| IBIS file stm32l4r5_s5_r7_s7_lqfp100.ibs
[IBIS ver]   4.2
[File name]   stm32l4r5_s5_r7_s7_lqfp100.ibs
[File Rev]   1.0
[Date]   01-6-2017
[Source]   Data Created at STMicroelectronics
[Notes]   File originated from ELDO simulations.
[Disclaimer]  This information is for modeling purpose only and is
   not guaranted.
   The information is subject to change without notice.
[Copyright]   Copyright 2017 STMicroelectronics Inc.
|   Component stm32l4r5_s5_r7_s7_lqfp100
[Component] stm32l4r5_s5_r7_s7_lqfp100
[Manufacturer] STMicroelectronics
[Package]
| variable   typ   min   max
R_pkg   0.0   0.0   0.0
L_pkg   0.0H   0.0H   0.0H
C_pkg   0.0F   0.0F   0.0F
[Pin]  signal_name   model_name   R_pin   L_pin   C_pin
1 PE2 io8prog2m25m50m120m_sudq_ft 132.430E-3 7.034E-9 135.000E-15
2 PE3 io8prog2m25m50m120m_sudq_ft 133.348E-3 6.765E-9 19.500E-15
3 PE4 io8prog2m25m50m120m_sudq_ft 128.973E-3 6.495E-9 10.400E-15
4 PE5 io8prog2m25m50m120m_sudq_ft 125.345E-3 6.206E-9 5.240E-15
5 PE6 io8prog2m25m50m120m_sudq_ft 120.515E-3 5.991E-9 7.820E-15
6 VBAT power 120.471E-3 5.950E-9 6.530E-15
7 PC13 io8prog2m25m50m120m_sudq_ft 117.881E-3 5.783E-9 6.230E-15
8 PC14-OSC32_IN io8prog2m25m50m120m_sudq_ft 117.279E-3 5.654E-9 3.110E-15
9 PC15-OSC32_OUT io8prog2m25m50m120m_sudq_ft 115.548E-3 5.548E-9 1.390E-15
10 VSS gnd 114.996E-3 5.434E-9 2.920E-15
11 VDD power 112.976E-3 5.296E-9 3.560E-15
12 PH0-OSC_IN io8prog2m25m50m120m_sudq_ft 111.323E-3 5.231E-9 4.780E-15
13 PH1-OSC_OUT io8prog2m25m50m120m_sudq_ft 109.217E-3 5.142E-9 8.660E-15
14 NRST ioreset_ft_v33 110.664E-3 5.180E-9 9.030E-15
15 PC0 io8prog2m25m50m120m_sudq_i2c_ft 110.608E-3 5.192E-9 7.980E-15
16 PC1 io8prog2m25m50m120m_sudq_i2c_ft 111.326E-3 5.252E-9 10.300E-15
17 PC2 io8prog2m25m50m120m_sudq_ft 114.420E-3 5.345E-9 7.000E-15
18 PC3 io8prog2m25m50m120m_sudq_ft 114.363E-3 5.454E-9 8.650E-15
19 VSSA gnd 117.564E-3 5.621E-9 7.825E-15
20 VREF- gnd 119.905E-3 5.800E-9 229.000E-18
21 VREF+ power 122.312E-3 5.963E-9 1.050E-15
22 VDDA power 125.384E-3 6.187E-9 812.000E-18
23 PA0 io8prog2m25m50m120m_sudq_ft 129.702E-3 6.485E-9 3.820E-15
24 PA1 io8prog2m25m50m120m_sudq_ft 132.290E-3 6.715E-9 6.800E-15
25 PA2 io8prog2m25m50m120m_sudq_ft 132.955E-3 7.014E-9 16.700E-15
26 PA3 io8prog2m25m50m120m_sudq_ft 133.943E-3 7.050E-9 17.500E-15
27 VSS gnd 134.958E-3 6.804E-9 12.700E-15
28 VDD power 130.511E-3 6.528E-9 9.830E-15
29 PA4 io8prog2m25m50m120m_sudq_ft 125.387E-3 6.245E-9 6.070E-15
30 PA5 io8prog2m25m50m120m_sudq_ft 124.989E-3 6.108E-9 577.000E-18
31 PA6 io8prog2m25m50m120m_sudq_ft 121.784E-3 5.890E-9 1.520E-15
32 PA7 io8prog2m25m50m120m_sudq_i2c_ft 119.149E-3 5.716E-9 5.440E-15
33 PC4 io8prog2m25m50m120m_sudq_ft 116.375E-3 5.556E-9 4.100E-15
34 PC5 io8prog2m25m50m120m_sudq_ft 113.279E-3 5.415E-9 3.690E-15
35 PB0 io8prog2m25m50m120m_sudq_ft 112.727E-3 5.358E-9 3.895E-15
36 PB1 io8prog2m25m50m120m_sudq_ft 112.271E-3 5.272E-9 1.660E-15
37 PB2 io8prog2m25m50m120m_sudq_ft 111.816E-3 5.238E-9 7.920E-15
38 PE7 io8prog2m25m50m120m_sudq_ft 110.999E-3 5.184E-9 9.900E-15
39 PE8 io8prog2m25m50m120m_sudq_ft 114.589E-3 5.299E-9 7.910E-15
40 PE9 io8prog2m25m50m120m_sudq_ft 114.461E-3 5.333E-9 7.940E-15
41 PE10 io8prog2m25m50m120m_sudq_ft 115.350E-3 5.424E-9 4.180E-15
42 PE11 io8prog2m25m50m120m_sudq_ft 116.979E-3 5.533E-9 6.060E-15
43 PE12 io8prog2m25m50m120m_sudq_ft 120.185E-3 5.698E-9 5.120E-15
44 PE13 io8prog2m25m50m120m_sudq_ft 122.587E-3 5.871E-9 4.740E-15
45 PE14 io8prog2m25m50m120m_sudq_ft 126.303E-3 6.069E-9 11.600E-15
46 PE15 io8prog2m25m50m120m_sudq_ft 129.715E-3 6.277E-9 9.910E-15
47 PB10 io8prog2m25m50m120m_sudq_i2c_ft 133.373E-3 6.508E-9 5.080E-15
48 PB11 io8prog2m25m50m120m_sudq_i2c_ft 137.888E-3 6.857E-9 5.470E-15
49 VSS gnd 131.554E-3 6.802E-9 4.180E-15
50 VDD power 132.348E-3 7.042E-9 11.900E-15
51 PB12 io8prog2m25m50m120m_sudq_ft 131.768E-3 7.008E-9 16.200E-15
52 PB13 io8prog2m25m50m120m_sudq_i2c_ft 131.784E-3 6.751E-9 2.150E-15
53 PB14 io8prog2m25m50m120m_sudq_i2c_ft 129.151E-3 6.483E-9 9.175E-15
54 PB15 io8prog2m25m50m120m_sudq_ft 125.191E-3 6.202E-9 5.663E-15
55 PD8 io8prog2m25m50m120m_sudq_ft 121.530E-3 5.986E-9 3.690E-15
56 PD9 io8prog2m25m50m120m_sudq_ft 118.874E-3 5.807E-9 7.430E-15
57 PD10 io8prog2m25m50m120m_sudq_ft 115.870E-3 5.635E-9 10.600E-15
58 PD11 io8prog2m25m50m120m_sudq_ft 113.226E-3 5.471E-9 5.760E-15
59 PD12 io8prog2m25m50m120m_sudq_ft 111.782E-3 5.354E-9 6.530E-15
60 PD13 io8prog2m25m50m120m_sudq_ft 110.713E-3 5.276E-9 11.400E-15
61 PD14 io8prog2m25m50m120m_sudq_ft 110.052E-3 5.204E-9 13.200E-15
62 PD15 io8prog2m25m50m120m_sudq_ft 109.954E-3 5.180E-9 14.600E-15
63 PC6 io8prog2m25m50m120m_sudq_ft 109.780E-3 5.154E-9 7.250E-15
64 PC7 io8prog2m25m50m120m_sudq_ft 112.446E-3 5.258E-9 359.000E-18
65 PC8 io8prog2m25m50m120m_sudq_ft 113.596E-3 5.332E-9 658.000E-18
66 PC9 io8prog2m25m50m120m_sudq_ft 115.707E-3 5.466E-9 508.500E-18
67 PA8 io8prog2m25m50m120m_sudq_ft 116.952E-3 5.598E-9 583.250E-18
68 PA9 power 119.043E-3 5.762E-9 545.875E-18
69 PA10 io8usb_id_otg20_lcd4_ft_ms 120.674E-3 5.880E-9 13.900E-15
70 PA11 io8usblsfs_otg2 124.659E-3 6.108E-9 25.000E-15
71 PA12 io8usblsfs_otg2 124.407E-3 6.161E-9 39.900E-15
72 PA13 io8prog2m25m50m120m_sudq_ft 130.156E-3 6.404E-9 302.000E-15
73 VDDUSB power 135.110E-3 6.824E-9 155.000E-15
74 VSS gnd 139.402E-3 7.077E-9 155.000E-15
75 VDD gnd 133.554E-3 7.056E-9 39.000E-15
76 PA14 io8prog2m25m50m120m_sudq_ft 135.295E-3 7.104E-9 16.300E-15
77 PA15 io8prog2m25m50m120m_sudq_ft 132.514E-3 6.836E-9 9.760E-15
78 PC10 io8prog2m25m50m120m_sudq_ft 133.482E-3 6.641E-9 9.300E-15
79 PC11 io8prog2m25m50m120m_sudq_ft 128.366E-3 6.341E-9 5.420E-15
80 PC12 io8prog2m25m50m120m_sudq_ft 124.282E-3 6.092E-9 1.180E-15
81 PD0 io8prog2m25m50m120m_sudq_ft 121.841E-3 5.917E-9 5.460E-15
82 PD1 io8prog2m25m50m120m_sudq_ft 118.487E-3 5.728E-9 7.000E-15
83 PD2 io8prog2m25m50m120m_sudq_ft 117.180E-3 5.573E-9 6.060E-15
84 PD3 io8prog2m25m50m120m_sudq_ft 113.501E-3 5.422E-9 5.450E-15
85 PD4 io8prog2m25m50m120m_sudq_ft 113.789E-3 5.344E-9 529.000E-18
86 PD5 io8prog2m25m50m120m_sudq_ft 110.806E-3 5.256E-9 2.990E-15
87 PD6 io8prog2m25m50m120m_sudq_ft 110.442E-3 5.246E-9 2.060E-15
88 PD7 io8prog2m25m50m120m_sudq_ft 111.525E-3 5.178E-9 5.680E-15
89 PB3 io8prog2m25m50m120m_sudq_ft 111.144E-3 5.223E-9 9.910E-15
90 PB4 io8prog2m25m50m120m_sudq_i2c_ft 113.222E-3 5.310E-9 9.050E-15
91 PB5 io8prog2m25m50m120m_sudq_ft 113.323E-3 5.401E-9 12.900E-15
92 PB6 io8prog2m25m50m120m_sudq_i2c_ft 115.849E-3 5.519E-9 12.600E-15
93 PB7 io8prog2m25m50m120m_sudq_i2c_ft 117.578E-3 5.673E-9 6.140E-15
94 PH3-BOOT0 io8prog2m25m50m120m_sudq_ft 118.982E-3 5.802E-9 9.370E-15
95 PB8 io8prog2m25m50m120m_sudq_i2c_ft 121.886E-3 5.962E-9 7.755E-15
96 PB9 io8prog2m25m50m120m_sudq_i2c_ft 126.276E-3 6.158E-9 8.563E-15
97 PE0 io8prog2m25m50m120m_sudq_ft 128.749E-3 6.367E-9 8.159E-15
98 PE1 io8prog2m25m50m120m_sudq_ft 133.288E-3 6.700E-9 1.030E-15
99 VSS gnd 132.230E-3 6.844E-9 4.410E-15
100 VDD power 132.277E-3 7.052E-9 17.100E-15
[Diff Pin]   inv_pin   vdiff   tdelay_typ  tdelay_min  tdelay_max
70 71 200mV   NA   NA   NA
[Model Selector] io8prog2m25m50m120m_sudq_ft
io8p00_sudq_ft_pd_lv  "SPEED00, PD=40kOhm - 1P8V"
io8p00_sudq_ft_pu_lv  "SPEED00, PU=40kOhm - 1P8V"
io8p00_sudq_ft_lv  "SPEED00 - 1P8V"
io8p00_sudq_ft_pd  "SPEED00, PD=40kOhm - 3P3V"
io8p00_sudq_ft_pu  "SPEED00, PU=40kOhm - 3P3V"
io8p00_sudq_ft  "SPEED00 - 3P3V"
io8p01_sudq_ft_pd_lv  "SPEED01, PD=40kOhm - 1P8V"
io8p01_sudq_ft_pu_lv  "SPEED01, PU=40kOhm - 1P8V"
io8p01_sudq_ft_lv  "SPEED01 - 1P8V"
io8p01_sudq_ft_pd  "SPEED01, PD=40kOhm - 3P3V"
io8p01_sudq_ft_pu  "SPEED01, PU=40kOhm - 3P3V"
io8p01_sudq_ft  "SPEED01 - 3P3V"
io8p10_sudq_ft_pd_lv  "SPEED10, PD=40kOhm - 1P8V"
io8p10_sudq_ft_pu_lv  "SPEED10, PU=40kOhm - 1P8V"
io8p10_sudq_ft_lv  "SPEED10 - 1P8V"
io8p10_sudq_ft_pd  "SPEED10, PD=40kOhm - 3P3V"
io8p10_sudq_ft_pu  "SPEED10, PU=40kOhm - 3P3V"
io8p10_sudq_ft  "SPEED10 - 3P3V"
io8p11_sudq_ft_pd_lv  "SPEED11, PD=40kOhm - 1P8V"
io8p11_sudq_ft_pu_lv  "SPEED11, PU=40kOhm - 1P8V"
io8p11_sudq_ft_lv  "SPEED11 - 1P8V"
io8p11_sudq_ft_pd  "SPEED11, PD=40kOhm - 3P3V"
io8p11_sudq_ft_pu  "SPEED11, PU=40kOhm - 3P3V"
io8p11_sudq_ft  "SPEED11 - 3P3V"
[Model Selector] io8prog2m25m50m120m_sudq_i2c_ft
io8prog_1v8_i2c_pd  "5V Tol GPIO 1.8V range i2c functionality with pull down"
io8prog_1v8_i2c_pu  "5V Tol GPIO 1.8V range i2c functionality with pull up"
io8prog_1v8_i2c  "5V Tol GPIO 1.8V range i2c functionality"
io8prog_3v3_i2c_pd  "5V Tol GPIO 3.3V range i2c functionality with pull down"
io8prog_3v3_i2c_pu  "5V Tol GPIO 3.3V range i2c functionality with pull up"
io8prog_3v3_i2c  "5V Tol GPIO 3.3V range i2c functionality"
io8prog_1v8_pd_00  "5V Tol GPIO 1.8V range with pd speed 00"
io8prog_1v8_pu_00  "5V Tol GPIO 1.8V range with pu speed 00"
io8prog_1v8_00  "5V Tol GPIO 1.8V range speed 00"
io8prog_3v3_pd_00  "5V Tol GPIO 3.3V range with pd speed 00"
io8prog_3v3_pu_00  "5V Tol GPIO 3.3V range with pu speed 00"
io8prog_3v3_00  "5V Tol GPIO 3.3V range speed 00"
io8prog_1v8_pd_01  "5V Tol GPIO 1.8V range with pd speed 01"
io8prog_1v8_pu_01  "5V Tol GPIO 1.8V range with pu speed 01"
io8prog_1v8_01  "5V Tol GPIO 1.8V range speed 01"
io8prog_3v3_pd_01  "5V Tol GPIO 3.3V range with pd speed 01"
io8prog_3v3_pu_01  "5V Tol GPIO 3.3V range with pu speed 01"
io8prog_3v3_01  "5V Tol GPIO 3.3V range speed 01"
io8prog_1v8_pd_10  "5V Tol GPIO 1.8V range with pd speed 10"
io8prog_1v8_pu_10  "5V Tol GPIO 1.8V range with pu speed 10"
io8prog_1v8_10  "5V Tol GPIO 1.8V range speed 10"
io8prog_3v3_pd_10  "5V Tol GPIO 3.3V range with pd speed 10"
io8prog_3v3_pu_10  "5V Tol GPIO 3.3V range with pu speed 10"
io8prog_3v3_10  "5V Tol GPIO 3.3V range speed 10"
io8prog_1v8_pd_11  "5V Tol GPIO 1.8V range with pd speed 11"
io8prog_1v8_pu_11  "5V Tol GPIO 1.8V range with pu speed 11"
io8prog_1v8_11  "5V Tol GPIO 1.8V range speed 11"
io8prog_3v3_pd_11  "5V Tol GPIO 3.3V range with pd speed 11"
io8prog_3v3_pu_11  "5V Tol GPIO 3.3V range with pu speed 11"
io8prog_3v3_11  "5V Tol GPIO 3.3V range speed 11"
[Model Selector] io8usb_id_otg20_lcd4_ft_ms
io8usbid_1v8_id_pu  "ID 1V8 range with pull up"
io8usbid_3v3_id_pu  "ID 3V3 range with pull up"
io8usbid_1v8_id  "ID 1V8 range"
io8usbid_3v3_id  "ID 3V3 range"
io8usbid_1v8_pd_00  "GPIO 1.8V range with pd speed 00"
io8usbid_1v8_pu_00  "GPIO 1.8V range with pu speed 00"
io8usbid_1v8_00  "GPIO 1.8V range speed 00"
io8usbid_3v3_pd_00  "GPIO 3.3V range with pd speed 00"
io8usbid_3v3_pu_00  "GPIO 3.3V range with pu speed 00"
io8usbid_3v3_00  "GPIO 3.3V range speed 00"
io8usbid_1v8_pd_01  "GPIO 1.8V range with pd speed 01"
io8usbid_1v8_pu_01  "GPIO 1.8V range with pu speed 01"
io8usbid_1v8_01  "GPIO 1.8V range speed 01"
io8usbid_3v3_pd_01  "GPIO 3.3V range with pd speed 01"
io8usbid_3v3_pu_01  "GPIO 3.3V range with pu speed 01"
io8usbid_3v3_01  "GPIO 3.3V range speed 01"
io8usbid_1v8_pd_10  "GPIO 1.8V range with pd speed 10"
io8usbid_1v8_pu_10  "GPIO 1.8V range with pu speed 10"
io8usbid_1v8_10  "GPIO 1.8V range speed 10"
io8usbid_3v3_pd_10  "GPIO 3.3V range with pd speed 10"
io8usbid_3v3_pu_10  "GPIO 3.3V range with pu speed 10"
io8usbid_3v3_10  "GPIO 3.3V range speed 10"
io8usbid_1v8_pd_11  "GPIO 1.8V range with pd speed 11"
io8usbid_1v8_pu_11  "GPIO 1.8V range with pu speed 11"
io8usbid_1v8_11  "GPIO 1.8V range speed 11"
io8usbid_3v3_pd_11  "GPIO 3.3V range with pd speed 11"
io8usbid_3v3_pu_11  "GPIO 3.3V range with pu speed 11"
io8usbid_3v3_11  "GPIO 3.3V range speed 11"
[Model Selector] io8usblsfs_otg2
usb_ls_pd  "USB Low Speed mode - Pull Down"
usb_ls_pu2  "USB Low Speed mode - Pull up 2"
usb_ls_pu  "USB Low Speed mode - Pull up"
usb_fs  "USB Low Speed mode"
usb_fs_pd  "USB Full Speed mode - Pull Down"
usb_fs_pu2  "USB Full Speed mode - Pull up 2"
usb_fs_pu  "USB Full Speed mode - Pull up"
[Model Selector] ioreset_ft_v33
ioreset_1v2_pu  "RESET 1.2V range with PU"
ioreset_1v2  "RESET 1.2V range"
ioreset_1v8_pu  "RESET 1.8V range with PU"
ioreset_1v8  "RESET 1.8V range"
ioreset_3v3_pu  "RESET 3.3V range with PU"
ioreset_3v3  "RESET 3.3V range"
| Models and submodels in the file (95): io8p00_sudq_ft_pd_lv (I/O), io8p00_sudq_ft_pu_lv (I/O), io8p00_sudq_ft_lv (I/O), io8p00_sudq_ft_pd (I/O), io8p00_sudq_ft_pu (I/O), io8p00_sudq_ft (I/O), io8p01_sudq_ft_pd_lv (I/O), io8p01_sudq_ft_pu_lv (I/O), io8p01_sudq_ft_lv (I/O), io8p01_sudq_ft_pd (I/O), io8p01_sudq_ft_pu (I/O), io8p01_sudq_ft (I/O), io8p10_sudq_ft_pd_lv (I/O), io8p10_sudq_ft_pu_lv (I/O), io8p10_sudq_ft_lv (I/O), io8p10_sudq_ft_pd (I/O), io8p10_sudq_ft_pu (I/O), io8p10_sudq_ft (I/O), io8p11_sudq_ft_pd_lv (I/O), io8p11_sudq_ft_pu_lv (I/O), io8p11_sudq_ft_lv (I/O), io8p11_sudq_ft_pd (I/O), io8p11_sudq_ft_pu (I/O), io8p11_sudq_ft (I/O), io8prog_1v8_i2c_pd (I/O), io8prog_1v8_i2c_pu (I/O), io8prog_1v8_i2c (I/O), io8prog_3v3_i2c_pd (I/O), io8prog_3v3_i2c_pu (I/O), io8prog_3v3_i2c (I/O), io8prog_1v8_pd_00 (I/O), io8prog_1v8_pu_00 (I/O), io8prog_1v8_00 (I/O), io8prog_3v3_pd_00 (I/O), io8prog_3v3_pu_00 (I/O), io8prog_3v3_00 (I/O), io8prog_1v8_pd_01 (I/O), io8prog_1v8_pu_01 (I/O), io8prog_1v8_01 (I/O), io8prog_3v3_pd_01 (I/O), io8prog_3v3_pu_01 (I/O), io8prog_3v3_01 (I/O), io8prog_1v8_pd_10 (I/O), io8prog_1v8_pu_10 (I/O), io8prog_1v8_10 (I/O), io8prog_3v3_pd_10 (I/O), io8prog_3v3_pu_10 (I/O), io8prog_3v3_10 (I/O), io8prog_1v8_pd_11 (I/O), io8prog_1v8_pu_11 (I/O), io8prog_1v8_11 (I/O), io8prog_3v3_pd_11 (I/O), io8prog_3v3_pu_11 (I/O), io8prog_3v3_11 (I/O), io8usbid_1v8_id_pu (Input), io8usbid_3v3_id_pu (Input), io8usbid_1v8_id (Input), io8usbid_3v3_id (Input), io8usbid_1v8_pd_00 (I/O), io8usbid_1v8_pu_00 (I/O), io8usbid_1v8_00 (I/O), io8usbid_3v3_pd_00 (I/O), io8usbid_3v3_pu_00 (I/O), io8usbid_3v3_00 (I/O), io8usbid_1v8_pd_01 (I/O), io8usbid_1v8_pu_01 (I/O), io8usbid_1v8_01 (I/O), io8usbid_3v3_pd_01 (I/O), io8usbid_3v3_pu_01 (I/O), io8usbid_3v3_01 (I/O), io8usbid_1v8_pd_10 (I/O), io8usbid_1v8_pu_10 (I/O), io8usbid_1v8_10 (I/O), io8usbid_3v3_pd_10 (I/O), io8usbid_3v3_pu_10 (I/O), io8usbid_3v3_10 (I/O), io8usbid_1v8_pd_11 (I/O), io8usbid_1v8_pu_11 (I/O), io8usbid_1v8_11 (I/O), io8usbid_3v3_pd_11 (I/O)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
